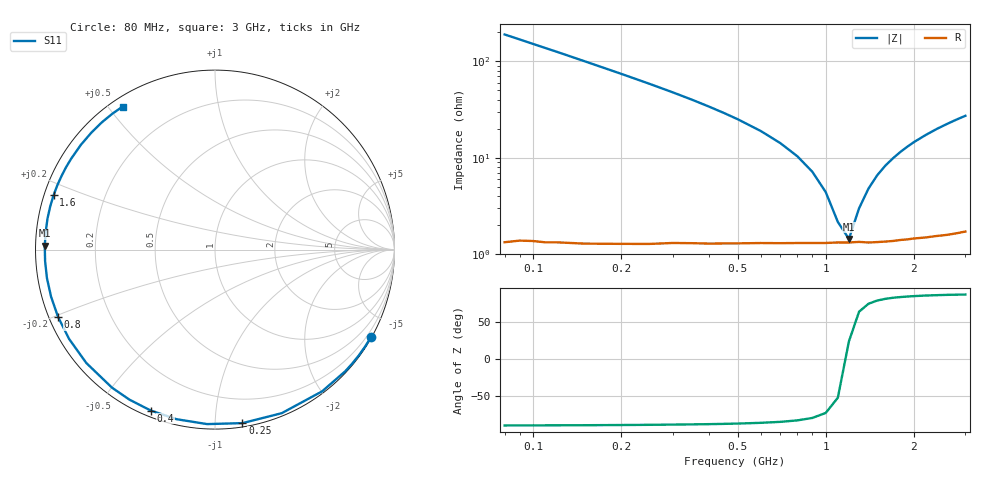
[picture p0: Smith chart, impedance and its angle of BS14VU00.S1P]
! SIEMENS Small Signal Semiconductors
! BB640
! Si Tuning Diode in SOD323
! VR = 14 V
! S-Parameters:  July  1993
# GHz  S  MA  R  50
!  f  S11
! GHz  MAG  ANG
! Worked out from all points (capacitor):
!   33 points, 80 MHz to 3 GHz, reference 50 ohm
!   read as one part to ground: C = 10.4 pF near 80 MHz
!   lowest |Z| = 1.43 ohm at 1.2 GHz (marker M1)
!   series resonance near 1.175 GHz, so ESL is about 1.8 nH
!   S11 on the Smith chart (normalised r, x): 80 MHz: 0.03, -3.81; 250 MHz: 0.03, -1.17; 400 MHz: 0.03, -0.68; 800 MHz: 0.03, -0.21; 1.6 GHz: 0.03, +0.16; 3 GHz: 0.03, +0.54
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0.08  0.9966 -29.4
0.11  0.9939 -39.8
0.12  0.9929 -43.1
0.15  0.9899 -52.9
0.2  0.9843 -67.8
0.25  0.9788 -81.0
0.3  0.9732 -92.6
0.35  0.9689 -102.8
0.4  0.9655 -111.8
0.45  0.9623 -119.7
0.5  0.9597 -126.7
0.6  0.9556 -138.6
0.7  0.9532 -148.5
0.8  0.9514 -156.8
0.9  0.9503 -164.0
1  0.9497 -170.4
1.1  0.9488 -176.1
1.2  0.9488 178.7
1.3  0.9482 173.9
1.4  0.9492 169.5
1.6  0.949 161.4
1.8  0.9483 154.3
2  0.948 147.8
2.2  0.9483 142.0
2.4  0.9483 136.6
2.6  0.9488 131.7
2.8  0.9488 127.1
3  0.9486 122.9
